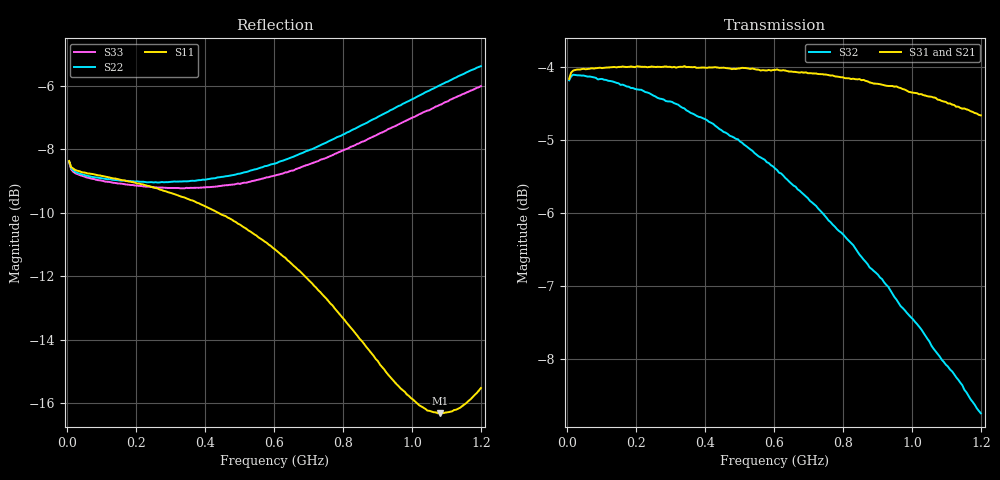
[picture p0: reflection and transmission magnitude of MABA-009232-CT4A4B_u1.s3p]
#	MHz	S	dB	R	50
!FREQ	R1	I1	R2	I2	R3	I3
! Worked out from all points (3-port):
!   201 points, 5 MHz to 1.2 GHz, reference 50 ohm
!   strongest paths, dB at 5 MHz, 303.8 MHz, 602.5 MHz, 901.2 MHz, 1.2 GHz:
!     S31: -4.2, -4.0, -4.0, -4.2, -4.7
!     S21: -4.2, -4.0, -4.1, -4.4, -4.9
!     S32: -4.2, -4.5, -5.4, -6.8, -8.8
!   lowest |S11| = -16.3 dB at 1.081 GHz (marker M1), VSWR 1.36, Z = 59.9 + j13.7 ohm
!   |S11| at or under -10 dB: 437.5 MHz to end of sweep
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5  -8.37 174.4  -4.16 -177.3  -4.16 2.7
   -4.16 -177.3  -8.38 173.6  -4.19 -177.7
   -4.16 2.7  -4.18 -177.8  -8.42 173.4
34.875  -8.70 176.3  -4.04 177.6  -4.03 -2.0
        -4.04 177.6  -8.77 171.6  -4.11 175.1
        -4.03 -2.0  -4.11 175.1  -8.81 171.2
154.375  -8.97 169.2  -4.03 166.7  -4.00 -11.6
         -4.03 166.7  -8.99 149.7  -4.23 156.7
         -4.00 -11.6  -4.24 156.6  -9.08 148.4
321.675  -9.46 158.0  -4.05 152.0  -4.00 -24.6
         -4.03 152.0  -9.02 118.5  -4.54 131.8
         -4.00 -24.6  -4.52 131.8  -9.22 116.0
453.125  -10.09 148.1  -4.08 140.5  -4.01 -35.0
         -4.10 140.4  -8.87 93.9  -4.87 112.7
         -4.01 -35.0  -4.89 112.7  -9.15 90.7
602.5  -11.16 134.5  -4.14 127.5  -4.04 -46.9
       -4.13 127.3  -8.46 66.7  -5.37 91.6
       -4.04 -46.9  -5.39 91.4  -8.83 62.6
841.5  -13.87 103.2  -4.30 106.7  -4.17 -66.5
       -4.32 106.3  -7.32 27.4  -6.49 59.2
       -4.17 -66.5  -6.53 58.9  -7.83 22.4
955.025  -15.39 80.5  -4.42 96.7  -4.27 -76.1
         -4.49 96.4  -6.68 11.2  -7.13 44.6
         -4.27 -76.1  -7.19 44.5  -7.25 6.2
1080.5  -16.31 47.1  -4.61 86.0  -4.45 -86.8
        -4.69 86.0  -5.99 -4.6  -7.91 29.5
        -4.45 -86.8  -7.97 29.7  -6.61 -9.7
1200  -15.52 13.4  -4.84 75.9  -4.66 -96.9
      -4.91 76.1  -5.39 -17.8  -8.68 15.8
      -4.66 -96.9  -8.75 16.2  -6.02 -22.9
